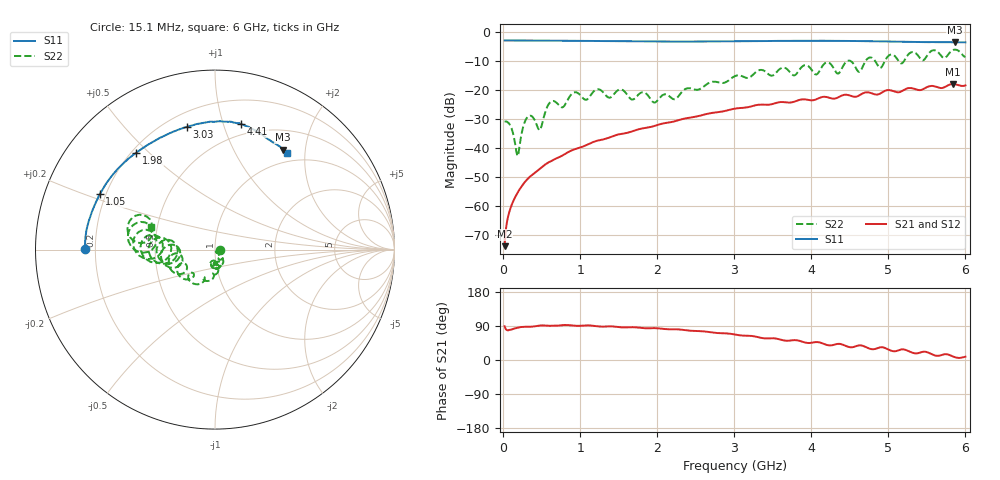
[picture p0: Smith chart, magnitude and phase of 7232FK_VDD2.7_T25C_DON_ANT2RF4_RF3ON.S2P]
!Agilent Technologies,E5071C,MY46417908,A.11.23
!Date: Fri Mar 03 11:30:47 2017
!Data & Calibration Information:
!Freq	S11:SOLT2(ON)	S21:SOLT2(ON)	S12:SOLT2(ON)	S22:SOLT2(ON)
!PortZ  Port1:50+j0  Port2:50+j0
!Above PortZ is port z conversion or system Z0 setting when saving the data.
!When reading, reference impedance value at option line is always used.
# Hz S dB R 50
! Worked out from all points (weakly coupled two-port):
!   400 points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, 15.1 MHz to 6 GHz, reference 50 ohm
!   highest |S21| = -17.86 dB at 5.835 GHz (marker M1); lowest = -73.8 dB at 15.1 MHz (marker M2)
!   lowest |S11| = -3.4 dB at 5.865 GHz (marker M3), VSWR 5.10, Z = 39.4 + j79.9 ohm
!   |S11| at or under -10 dB: nowhere
!   |S22| runs from -42.7 to -5.9 dB; largest |S21 - S12| = 0.0026
!   S11 on the Smith chart (normalised r, x): 15.1 MHz: 0.16, +0.00; 1.05 GHz: 0.18, +0.22; 1.98 GHz: 0.22, +0.46; 3.03 GHz: 0.28, +0.76; 4.41 GHz: 0.40, +1.15; 6 GHz: 0.84, +1.67
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1.509975e7  -2.78 179.6  -73.82 88.9  -73.71 89.6  -30.74 -8.3
6.0099e7  -2.79 178.6  -63.60 78.3  -63.59 78.9  -31.13 -34.9
1.80097e8  -2.79 175.8  -55.54 85.0  -55.52 85.0  -42.70 -42.8
3.150948e8  -2.80 172.9  -50.57 87.8  -50.56 87.8  -29.15 -35.8
4.650922e8  -2.82 169.7  -47.27 90.6  -47.28 90.7  -33.76 -58.1
6.150898e8  -2.86 166.1  -44.53 90.3  -44.53 90.4  -23.97 -46.2
1.020083e9  -2.94 155.1  -39.56 90.6  -39.58 90.5  -22.32 -82.3
1.050082e9  -2.95 154.3  -39.24 91.0  -39.27 91.0  -23.09 -80.1
1.515075e9  -3.04 141.5  -35.12 86.3  -35.13 86.4  -19.69 -92.6
1.980067e9  -3.15 129.0  -32.14 84.0  -32.14 84.0  -24.04 -90.6
2.010066e9  -3.16 128.1  -31.89 83.6  -31.90 83.6  -23.23 -85.6
3.01505e9  -3.08 103.4  -26.29 66.9  -26.28 67.0  -15.01 -101.2
3.03005e9  -3.08 103.1  -26.22 66.4  -26.21 66.4  -14.88 -103.6
4.005033e9  -2.90 84.4  -23.46 45.6  -23.44 45.5  -13.01 -174.6
4.410026e9  -2.93 78.3  -21.67 40.2  -21.65 40.1  -11.70 -162.8
4.620023e9  -2.98 74.8  -21.77 38.6  -21.75 38.5  -13.67 -178.5
4.77002e9  -3.05 72.9  -20.90 29.0  -20.87 29.0  -8.64 178.7
4.890018e9  -3.09 70.8  -21.17 33.3  -21.12 32.8  -12.28 177.7
5.010016e9  -3.15 70.0  -19.91 26.7  -19.85 26.8  -7.89 -175.3
5.835003e9  -3.43 56.6  -17.86 9.6  -17.80 10.6  -6.14 169.3
5.865002e9  -3.45 55.8  -17.93 7.3  -17.82 8.1  -5.94 164.1
6e9  -3.43 53.3  -18.30 8.6  -18.30 9.5  -8.50 160.3
